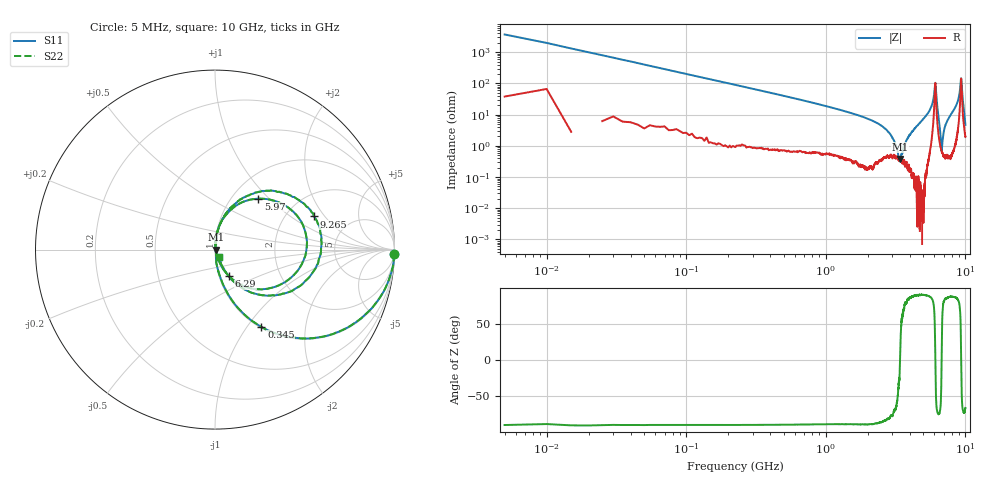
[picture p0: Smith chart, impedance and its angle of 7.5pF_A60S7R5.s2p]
! Amotech Co.,Ltd.
! http://www.amotech.co.kr/
! Part Number: A60S7R5
! These Parameters are Measured in Series Mode Connection
! Operation Temp=25[degC], DC Bias Voltage=0[V]
! Freq. Start=5[MHz] Stop=10[GHz], 2000[Steps]
! Date: Monday, July 13, 2020, 01:32:55
# GHZ S RI R 50.000000
!Freq.(Hz) S11(Real) S11(Imag) S21(Real) S21(Imag) S12(Real) S12(Imag) S22(Real) S22(Imag)
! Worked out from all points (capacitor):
!   2000 points, 5 MHz to 10 GHz, reference 50 ohm
!   read as one part in series: C = 7.87 pF near 55 MHz
!   lowest |Z| = 380 mohm at 3.4 GHz (marker M1)
!   series resonance near 3.402 GHz, so ESL is about 280 pH
!   S11 on the Smith chart (normalised r, x): 5 MHz: 2, -74; 345 MHz: 1.02, -1.17; 5.97 GHz: 1.31, +0.86; 6.29 GHz: 1.12, -0.34; 9.265 GHz: 2.81, +1.57; 10 GHz: 1.04, -0.09
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0.005  0.999 -0.0268  0.000996 0.0268  0.000996 0.0268  0.999 -0.0268
0.065  0.9036 -0.2886  0.0964 0.2886  0.0964 0.2886  0.9036 -0.2886
0.11  0.7683 -0.4153  0.2317 0.4153  0.2317 0.4153  0.7683 -0.4153
0.345  0.2587 -0.4305  0.7413 0.4305  0.7413 0.4305  0.2587 -0.4305
1.675  0.0124 -0.0967  0.9876 0.0967  0.9876 0.0967  0.0124 -0.0967
2.855  0.0052 -0.0251  0.9948 0.0251  0.9948 0.0251  0.0052 -0.0251
3.34  0.00379 -0.00203  0.9962 0.00203  0.9962 0.00203  0.00379 -0.00203
3.4  0.00378 -0.000252  0.9962 0.000252  0.9962 0.000252  0.00378 -0.000252
3.955  0.00236 0.0212  0.9976 -0.0212  0.9976 -0.0212  0.00236 0.0212
5.005  0.00543 0.0733  0.9946 -0.0733  0.9946 -0.0733  0.00543 0.0733
5.97  0.2405 0.2836  0.7595 -0.2836  0.7595 -0.2836  0.2405 0.2836
6.09  0.5083 -0.00801  0.4917 0.00801  0.4917 0.00801  0.5083 -0.00801
6.17  0.2762 -0.22  0.7238 0.22  0.7238 0.22  0.2762 -0.22
6.29  0.0796 -0.1489  0.9204 0.1489  0.9204 0.1489  0.0796 -0.1489
6.67  0.00853 -0.0131  0.9915 0.0131  0.9915 0.0131  0.00853 -0.0131
6.77  0.00642 0.0025  0.9936 -0.0025  0.9936 -0.0025  0.00642 0.0025
7.135  0.00563 0.0405  0.9944 -0.0405  0.9944 -0.0405  0.00563 0.0405
8.335  0.0305 0.1467  0.9695 -0.1467  0.9695 -0.1467  0.0305 0.1467
8.955  0.146 0.2813  0.854 -0.2813  0.854 -0.2813  0.146 0.2813
9.265  0.5511 0.1845  0.4489 -0.1845  0.4489 -0.1845  0.5511 0.1845
9.465  0.3319 -0.2556  0.6681 0.2556  0.6681 0.2556  0.3319 -0.2556
10  0.0206 -0.0413  0.9794 0.0413  0.9794 0.0413  0.0206 -0.0413
